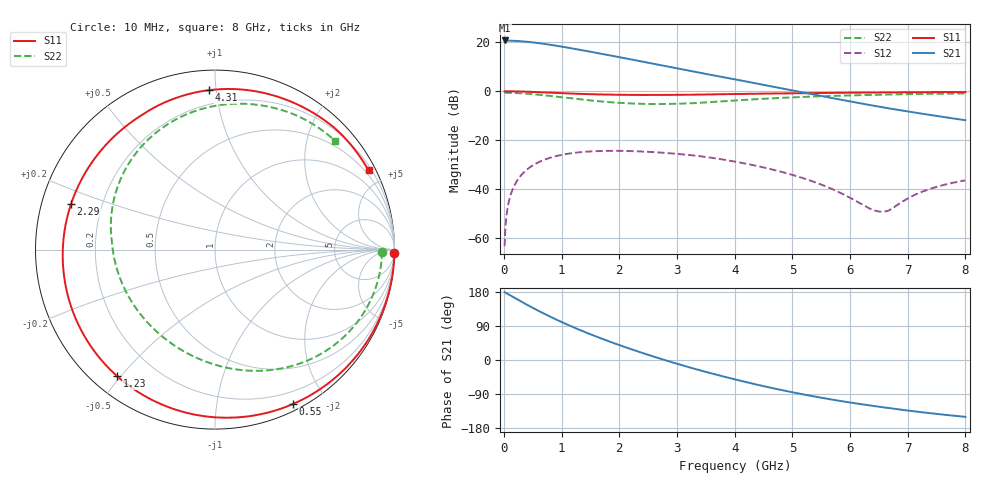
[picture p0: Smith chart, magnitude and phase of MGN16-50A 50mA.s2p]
! Port[1] = GATE
! Port[2] = DRAIN
! [Type]  S-parameter s2p file touchstone ver. 1.0
! [Object]  MGN16-50A
! [Bias]  50 mA
! [Version]  1.0
! [Date]  Thu May 28 10:54:03 2026
! [Source]  This file was created in JSC "ICC Milandr".
! [Disclaimer] Property of JSC "ICC Milandr". Unauthorized reproduction and/or distribution is strictly prohibited.
!  The file and the data are provided "AS IS" and with all faults and disclaim all warranties, express and implied, including
!  without limitation any implied warranties of merchantability, fitness for a particular purpose.
!  JSC "ICC Milandr" assumes no liability for:
!  1) the accuracy of the data provided;
!  2) the proper functioning of this data;
!  3) infringement of patents, copyrights or intellectual property rights resulting from the use of this data.
!  JSC "ICC Milandr" reserves the right to make changes to the products and the data without prior notice.
!  Please, be aware that your receipt and use of the file provided shall serve as acceptance of these terms and conditions.
!  If you do not accept these terms, you should return or destroy this file and any other accompanying information immediately.
# hz S ma R 12.5
! 2 Port Network Data from SP1.SP block
! freq  magS11  angS11  magS21  angS21  magS12  angS12  magS22  angS22
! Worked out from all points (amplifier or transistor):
!   800 points, 10 MHz to 8 GHz, reference 12.5 ohm
!   highest |S21| = 20.8 dB at 10 MHz (marker M1)
!   |S21| within 3 dB of that: start of sweep to 1.118 GHz
!   unconditionally stable (mu >= 1): 4.39 GHz to end of sweep
!   at 1.34 GHz: K = 0.18, MSG = 20.9 dB, |S12| = -24.9 dB
!   at 4.01 GHz: K = 0.81, MSG = 16.8 dB, |S12| = -28.8 dB
!   at 8 GHz: K = 1.63, MAG = 7.7 dB, |S12| = -36.5 dB
!   S11 on the Smith chart (normalised r, x): 10 MHz: 2, -97; 550 MHz: 0.07, -1.62; 1.23 GHz: 0.07, -0.49; 2.29 GHz: 0.09, +0.15; 4.31 GHz: 0.11, +0.96; 8 GHz: 0.34, +4.10
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1e7  0.9996 -1.2  10.99 179.1  0.0006717 82.6  0.9306 -0.7
1e8  0.9981 -12.0  10.92 171.2  0.00662 80.9  0.9279 -6.8
2.5e8  0.9908 -29.7  10.69 158.2  0.01621 68.9  0.9142 -16.8
4e8  0.9788 -46.8  10.33 145.6  0.02506 57.0  0.891 -26.6
5.5e8  0.9637 -63.3  9.865 133.5  0.03292 45.5  0.8608 -36.0
7e8  0.9469 -79.0  9.34 121.8  0.03967 34.4  0.8264 -44.9
8.6e8  0.9288 -94.9  8.746 110.0  0.04564 23.2  0.7878 -54.1
1.03e9  0.9104 -110.6  8.107 98.0  0.05066 11.8  0.747 -63.5
1.23e9  0.8913 -127.8  7.374 84.6  0.05499 -0.8  0.7018 -74.0
1.35e9  0.8813 -137.5  6.953 77.0  0.05689 -8.0  0.6769 -80.2
1.56e9  0.8666 -153.2  6.259 64.2  0.05911 -20.0  0.6383 -90.9
1.78e9  0.8551 -168.1  5.595 51.4  0.06019 -32.0  0.605 -102.1
2.02e9  0.8465 177.1  4.943 38.2  0.0602 -44.5  0.5774 -114.5
2.29e9  0.8413 162.4  4.295 24.1  0.05908 -57.8  0.5573 -128.6
2.68e9  0.8406 144.0  3.498 4.9  0.05586 -76.0  0.5476 -149.4
2.97e9  0.8443 132.2  2.996 -8.6  0.05259 -88.8  0.5539 -164.9
3.27e9  0.851 121.4  2.546 -21.8  0.04868 -101.5  0.5705 179.5
4.01e9  0.8788 99.8  1.749 -51.4  0.03616 -125.5  0.649 146.0
4.31e9  0.8891 92.1  1.497 -62.4  0.03084 -133.9  0.6822 133.9
5.34e9  0.9188 69.1  0.8701 -95.1  0.01443 -154.7  0.7784 98.7
6.67e9  0.9499 45.9  0.4468 -126.7  0.003592 -89.4  0.8587 65.9
8e9  0.9628 27.3  0.2554 -150.0  0.01497 -59.9  0.9025 42.1
